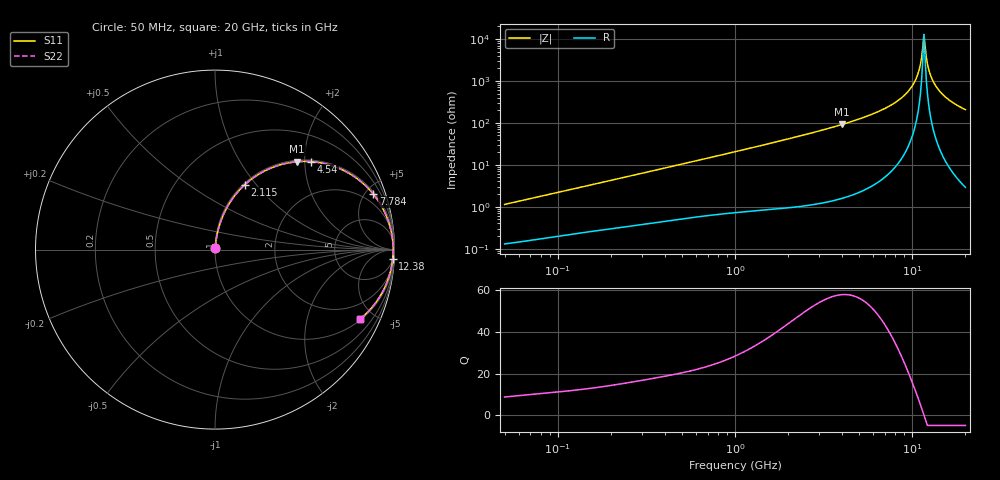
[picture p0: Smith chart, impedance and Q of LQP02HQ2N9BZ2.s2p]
!Murata Part Number: LQP02HQ2N9BZ2
!These Parameters are Measured in Series Mode Connection
!  o--[Z]--o
!Port1  Port2
!  o-------o
!Freq. Start=50[MHz] Stop=20[GHz], 401[Steps]
# Hz S RI R 50
!Freq.(Hz) S11(Real) S11(Imag) S21(Real) S21(Imag) S12(Real) S12(Imag) S22(Real) S22(Imag)
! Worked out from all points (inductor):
!   401 points, 50 MHz to 20 GHz, reference 50 ohm
!   read as one part in series: L = 3.55 nH near 51.52 MHz
!   highest Q = 58 at 4.027 GHz (marker M1), where L = 3.62 nH
!   self-resonance near 11.66 GHz
!   S11 on the Smith chart (normalised r, x): 50 MHz: 1.00, +0.02; 2.115 GHz: 1.02, +0.88; 4.54 GHz: 1.04, +2.15; 7.784 GHz: 1.15, +5.62; 12.38 GHz: 7, -39; 20 GHz: 1.06, -4.14
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5e7  0.00142 0.0112  0.9986 -0.0112  0.9986 -0.0112  0.00142 0.0112
1.364002e8  0.00324 0.0293  0.9968 -0.0293  0.9968 -0.0293  0.00324 0.0293
3.721004e8  0.0102 0.0765  0.9898 -0.0765  0.9898 -0.0765  0.0102 0.0765
1e9  0.0465 0.1936  0.9535 -0.1936  0.9535 -0.1936  0.0465 0.1936
2.114743e9  0.1675 0.3626  0.8325 -0.3626  0.8325 -0.3626  0.1675 0.3626
2.728004e9  0.2555 0.4267  0.7445 -0.4267  0.7445 -0.4267  0.2555 0.4267
4.026975e9  0.4575 0.4896  0.5425 -0.4896  0.5425 -0.4896  0.4575 0.4896
4.539627e9  0.5344 0.4902  0.4656 -0.4902  0.4656 -0.4902  0.5344 0.4902
7.442007e9  0.8572 0.3376  0.1428 -0.3376  0.1428 -0.3376  0.8572 0.3376
7.784049e9  0.881 0.3105  0.119 -0.3105  0.119 -0.3105  0.881 0.3105
9.178299e9  0.9512 0.1956  0.0488 -0.1956  0.0488 -0.1956  0.9512 0.1956
1.019291e10  0.9788 0.1128  0.0212 -0.1128  0.0212 -0.1128  0.9788 0.1128
1.082228e10  0.988 0.0634  0.012 -0.0634  0.012 -0.0634  0.988 0.0634
1.115139e10  0.9907 0.0383  0.00933 -0.0383  0.00933 -0.0383  0.9907 0.0383
1.131968e10  0.9915 0.0257  0.00847 -0.0257  0.00847 -0.0257  0.9915 0.0257
1.166392e10  0.9923 0.000546  0.00771 -0.000546  0.00771 -0.000546  0.9923 0.000546
1.201863e10  0.9918 -0.0247  0.00823 0.0247  0.00823 0.0247  0.9918 -0.0247
1.238412e10  0.99 -0.0498  0.01 0.0498  0.01 0.0498  0.99 -0.0498
1.314879e10  0.9825 -0.0996  0.0175 0.0996  0.0175 0.0996  0.9825 -0.0996
1.460232e10  0.9576 -0.1836  0.0424 0.1836  0.0424 0.1836  0.9576 -0.1836
1.670968e10  0.9053 -0.2818  0.0947 0.2818  0.0947 0.2818  0.9053 -0.2818
2e10  0.8074 -0.3874  0.1926 0.3874  0.1926 0.3874  0.8074 -0.3874
